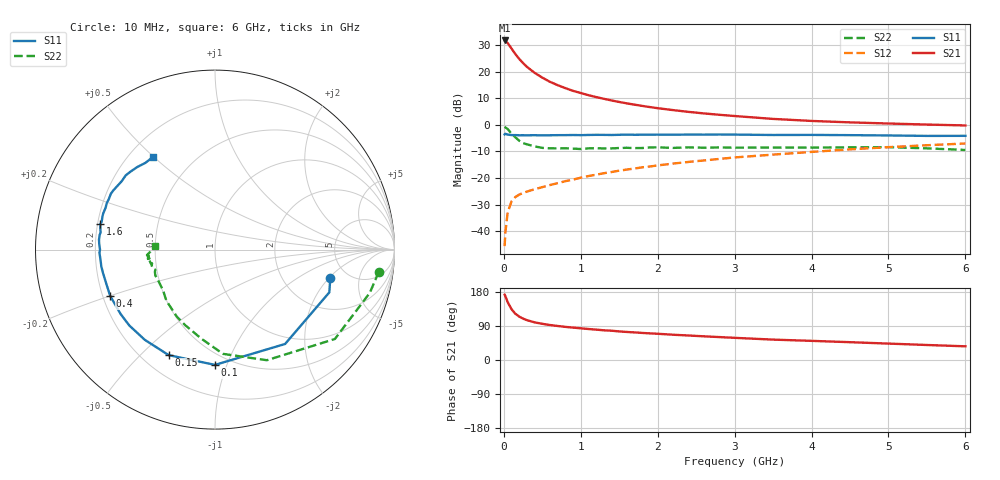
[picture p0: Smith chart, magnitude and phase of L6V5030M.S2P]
!  INFINEON TECHNOLOGIES Small Signal Semiconductors
! BFR380L3 , Si-NPN RF-Transistor in TSLP-3-1
!  Vce=0.5 V,  Ic=30 mA
! Common Emitter S-Parameters:  07. March 2005
#  GHz  S  MA  R  50
! f  S11  S21  S12  S22
! GHz  Mag  Ang  Mag  Ang  Mag  Ang  Mag  Ang
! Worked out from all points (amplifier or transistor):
!   36 points, 10 MHz to 6 GHz, reference 50 ohm
!   highest |S21| = 31.8 dB at 10 MHz (marker M1)
!   |S21| within 3 dB of that: start of sweep to 98.92 MHz
!   unconditionally stable (mu >= 1): 1.219 GHz to end of sweep
!   at 250 MHz: K = 0.48, MSG = 24.5 dB, |S12| = -25.7 dB
!   at 1.4 GHz: K = 1.03, MAG = 12.5 dB, |S12| = -17.8 dB
!   at 6 GHz: K = 1.01, MAG = 2.7 dB, |S12| = -7.0 dB
!   S11 on the Smith chart (normalised r, x): 10 MHz: 3.66, -2.08; 100 MHz: 0.42, -0.91; 150 MHz: 0.30, -0.61; 400 MHz: 0.23, -0.20; 1.6 GHz: 0.21, +0.10; 6 GHz: 0.30, +0.50
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0.01  0.6618 -14.0  38.83 172.3  0.0052 77.8  0.9208 -7.8
0.02  0.68 -20.5  38.21 168.5  0.0095 80.9  0.8956 -15.6
0.05  0.6549 -53.4  34.57 152.6  0.0225 68.1  0.8332 -36.7
0.1  0.6423 -90.0  27.35 134.0  0.0362 54.0  0.6806 -64.9
0.15  0.6421 -113.7  21.52 122.0  0.0438 47.3  0.5826 -85.6
0.2  0.637 -127.9  17.45 114.5  0.0487 44.9  0.5025 -98.6
0.25  0.6377 -138.4  14.57 109.2  0.052 43.4  0.4529 -111.4
0.3  0.6367 -145.7  12.38 105.2  0.0554 43.9  0.4303 -119.5
0.4  0.6385 -156.2  9.543 99.3  0.0614 45.4  0.3931 -133.6
0.5  0.6348 -163.3  7.744 95.5  0.0672 48.3  0.3688 -141.4
0.6  0.6373 -168.0  6.458 92.3  0.0737 50.2  0.3622 -147.3
0.7  0.6402 -171.5  5.59 89.8  0.0799 52.2  0.3603 -152.6
0.9  0.6441 -178.4  4.367 85.5  0.0932 55.5  0.3567 -159.9
1.1  0.6457 177.3  3.62 81.8  0.1088 57.8  0.3611 -162.8
1.3  0.6477 172.7  3.096 78.4  0.1229 59.0  0.3591 -167.8
1.6  0.6541 167.5  2.537 74.0  0.144 60.3  0.37 -170.8
2.2  0.6525 159.2  1.896 66.7  0.1866 61.1  0.3683 -172.3
2.8  0.6585 151.7  1.548 60.5  0.2282 61.1  0.3757 -175.4
3.5  0.6445 143.7  1.294 53.8  0.2753 58.8  0.3743 -175.3
4.5  0.6403 137.2  1.114 47.0  0.3455 56.2  0.3775 -175.6
5.5  0.6197 128.8  1.013 39.6  0.4134 51.4  0.361 -178.1
6  0.621 123.8  0.975 36.1  0.4461 48.9  0.3367 176.6
